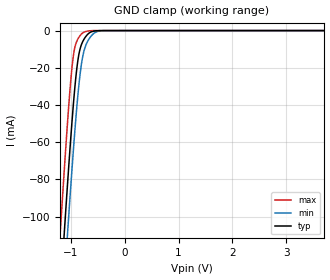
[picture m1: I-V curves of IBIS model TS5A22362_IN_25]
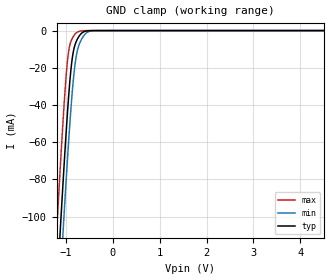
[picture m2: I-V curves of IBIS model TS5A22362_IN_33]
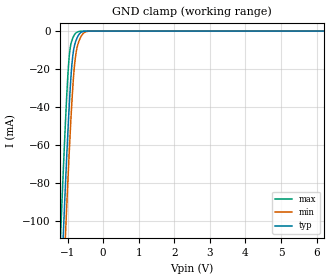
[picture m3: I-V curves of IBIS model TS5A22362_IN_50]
| TEXAS INSTRUMENTS INCORPORATED
| Standard Linear and Logic Group
| IBIS Model of TS5A22362
| 0.65-OHM DUAL SPDT ANALOG SWITCHES WITH NEGATIVE SIGNALING CAPABILITY
| This file contains package information for the following:
|  VSSOP 10-pin (DGS) package as [Component] TS5A22362_DGS
| This device can be powered at the following Vccs:
|  2.5 volt Vcc
|  3.3 volt Vcc
|  5 volt Vcc
| This file provides unique models under the [Model Selector] for each Vcc.
| For operation at a specific Vcc, select the appropriate model after each
| [Model Selector] keyword.
[IBIS Ver]   3.2
[Comment char]  |_char
[File Name]   ts5a22362.ibs
[File Rev]   1.0 | x_die
[Date]   March 22, 2009
[Source]   Data created from TI-SPICE simulations at TI-SLL.
[Notes]   The following is an IBIS list for the TS5A22362.
   Please contact sllibis@ti.com with questions and
   comments concerning SLL IBIS models.
   - FILE REV HISTORY
   - 1.0 Release IBIS file on 03/23/09.
   - Power clamp data deleted was deleted as there is no
   power-clamp diode.
   - No ground clamp current for the COM and N models
   due to negative voltages passed through the switch.
   - Non-monotonic data due to FET characteristics.
[Disclaimer] Property of Texas Instruments Incorporated.  Unauthorized
   reproduction and/or distribution is strictly prohibited.
   This product is protected under copyright law.
   Created  2009, (C) Copyright  2009, Texas Instruments
   Incorporated, All Rights Reserved
   UNLESS THERE IS A SIGNED, WRITTEN AGREEMENT TO THE
   CONTRARY, TEXAS INSTRUMENTS (TI) IS PROVIDING THE IBIS
   MODELS  AND WITHOUT ANY WARRANTY, EXPRESSED OR
   IMPLIED.  TI assumes no liability for:
   1) the accuracy of the IBIS models provided to your
   company;
   2) the proper functioning of these IBIS Models in your
   design or for any resulting applications; or
   3) infringement of patents, copyrights or intellectual
   property rights resulting from your use of these IBIS
   models.
   TI provides IBIS Models as a service to our customers.
   You and your company shall not distribute, sell or give
   these models to anyone else without prior written
   permission from TI.
   TI reserves the right to make changes to our products or
   to discontinue any semiconductor product or service
   without notice, and advises our customers to obtain the
   latest version of relevant information to verify, before
   placing orders, that the information being relied on is
   current.
   Please be aware that your receipt and use of the IBIS
   information provided shall serve as acceptance of these
   terms and conditions.  If you do not accept these terms,
   you should return or destroy the IBIS models and any
   other accompanying information immediately.
| Component TS5A22362_DGS 10-PIN VSSOP
[Component]   TS5A22362_DGS
[Manufacturer]   Texas Instruments, Inc.
[Package]
|   typ   min   max
R_pkg   4.300e-02   4.100e-02   4.700e-02
L_pkg   2.235e-09   2.157e-09   2.339e-09
C_pkg   3.350e-13   3.080e-13   3.550e-13
[Pin]   signal_name   model_name   R_pin   L_pin   C_pin
1   VP   POWER   4.700e-02   2.339e-09   3.100e-13
2   NO1   TS5A22362_N   4.300e-02   2.213e-09   3.550e-13
3   COM1   TS5A22362_COM   4.100e-02   2.157e-09   3.540e-13
4   NC1   TS5A22362_N   4.300e-02   2.213e-09   3.550e-13
5   IN1   TS5A22362_IN   4.700e-02   2.339e-09   3.100e-13
6   GND   GND   4.500e-02   2.284e-09   3.080e-13
7   IN2   TS5A22362_IN   4.100e-02   2.176e-09   3.500e-13
8   NC2   TS5A22362_N   4.100e-02   2.172e-09   3.500e-13
9   COM2   TS5A22362_COM   4.100e-02   2.176e-09   3.510e-13
10   NO2   TS5A22362_N   4.500e-02   2.284e-09   3.080e-13
[Series Switch Groups]
| Function Group States
On  1 /   | NC1-NC2->COM1-COM2 IN1-IN2, LOW
   | COM1-COM2->NC1-NC2 IN1-IN2, LOW
On  2 /   | NO1-NO2->COM1-COM2 IN1-IN2, HIGH
   | COM1-COM2->NO1-NO2 IN1-IN2, HIGH
On  1 /   | IN1-IN2, LOW
Off 2 /   | IN1-IN2, HIGH
[Series Pin Mapping]   pin_2   model_name   function_table_group
4   3   TS5A22362_N_25_S   1
| 4   3   TS5A22362_N_33_S   1
| 4   3   TS5A22362_N_50_S   1
8   9   TS5A22362_N_25_S   1
| 8   9   TS5A22362_N_33_S   1
| 8   9   TS5A22362_N_50_S   1
3   4   TS5A22362_COM_25_S   1
| 3   4   TS5A22362_COM_33_S   1
| 3   4   TS5A22362_COM_50_S   1
9   8   TS5A22362_COM_25_S   1
| 9   8   TS5A22362_COM_33_S   1
| 9   8   TS5A22362_COM_50_S   1
2   3   TS5A22362_N_25_S   2
| 2   3   TS5A22362_N_33_S   2
| 2   3   TS5A22362_N_50_S   2
10   9   TS5A22362_N_25_S   2
| 10   9   TS5A22362_N_33_S   2
| 10   9   TS5A22362_N_50_S   2
3   2   TS5A22362_COM_25_S   2
| 3   2   TS5A22362_COM_33_S   2
| 3   2   TS5A22362_COM_50_S   2
9   10   TS5A22362_COM_25_S   2
| 9   10   TS5A22362_COM_33_S   2
| 9   10   TS5A22362_COM_50_S   2
| Model TS5A22362_IN
[Model Selector]   TS5A22362_IN
TS5A22362_IN_25   2.5 volt Vcc
TS5A22362_IN_33   3.3 volt Vcc
TS5A22362_IN_50   5 volt Vcc
| Model TS5A22362_N
[Model Selector]   TS5A22362_N
TS5A22362_N_25   2.5 volt Vcc
TS5A22362_N_33   3.3 volt Vcc
TS5A22362_N_50   5 volt Vcc
| Model TS5A22362_N_S
[Model Selector]   TS5A22362_N_S
TS5A22362_N_25_S   2.5 volt Vcc
TS5A22362_N_33_S   3.3 volt Vcc
TS5A22362_N_50_S   5 volt Vcc
| Model TS5A22362_COM
[Model Selector]   TS5A22362_COM
TS5A22362_COM_25   2.5 volt Vcc
TS5A22362_COM_33   3.3 volt Vcc
TS5A22362_COM_50   5 volt Vcc
| Model TS5A22362_COM_S
[Model Selector]   TS5A22362_COM_S
TS5A22362_COM_25_S   2.5 volt Vcc
TS5A22362_COM_33_S   3.3 volt Vcc
TS5A22362_COM_50_S   5 volt Vcc
[Model]   TS5A22362_N_25_S
Model_type  Series_switch
| variable   typ   min   max
C_comp   0   0   0
[Temperature Range]   40   100   -40
| Ambient temperature   25   85   -40
[Voltage range]   2.5   2.3   2.7
[On]
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[Off]
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[Model]   TS5A22362_N_33_S
Model_type  Series_switch
| variable   typ   min   max
C_comp   0   0   0
[Temperature Range]   40   100   -40
| Ambient temperature   25   85   -40
[Voltage range]   3.3   3   3.6
[On]
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[Off]
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[Model]   TS5A22362_N_50_S
Model_type  Series_switch
| variable   typ   min   max
C_comp   0   0   0
[Temperature Range]   40   100   -40
| Ambient temperature   25   85   -40
[Voltage range]   5   4.5   5.5
[On]
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[Off]
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[Model]   TS5A22362_COM_25_S
Model_type  Series_switch
| variable   typ   min   max
C_comp   0   0   0
[Temperature Range]   40   100   -40
| Ambient temperature   25   85   -40
[Voltage range]   2.5   2.3   2.7
[On]
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[Off]
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[Model]   TS5A22362_COM_33_S
Model_type  Series_switch
| variable   typ   min   max
C_comp   0   0   0
[Temperature Range]   40   100   -40
| Ambient temperature   25   85   -40
[Voltage range]   3.3   3   3.6
[On]
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[Off]
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[Model]   TS5A22362_COM_50_S
Model_type  Series_switch
| variable   typ   min   max
C_comp   0   0   0
[Temperature Range]   40   100   -40
| Ambient temperature   25   85   -40
[Voltage range]   5   4.5   5.5
[On]
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[Off]
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| Models and submodels in the file (15): TS5A22362_IN_25 (Input), TS5A22362_IN_33 (Input), TS5A22362_IN_50 (Input), TS5A22362_N_25_S (Series_switch), TS5A22362_N_25 (Terminator), TS5A22362_N_33_S (Series_switch), TS5A22362_N_33 (Terminator), TS5A22362_N_50_S (Series_switch), TS5A22362_N_50 (Terminator), TS5A22362_COM_25_S (Series_switch), TS5A22362_COM_25 (Terminator), TS5A22362_COM_33_S (Series_switch), TS5A22362_COM_33 (Terminator), TS5A22362_COM_50_S (Series_switch), TS5A22362_COM_50 (Terminator)
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[Model]   TS5A22362_IN_25
Model_type  Input
Vinl=0.6
Vinh=1.4
| variable   typ   min   max
C_comp   2.05pF   1.68pF   2.72pF
[Temperature Range]   40   100   -40
| Ambient temperature   25   85   -40
[Voltage range]   2.5   2.3   2.7
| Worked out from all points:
|   GND clamp passes 1 mA (typ) near -0.64 V on its own axis
[GND Clamp]
| TS5A22362_IN_25
|   Voltage   I(typ)   I(min)   I(max)
-2.5V     -779mA     -802.6mA   -750.6mA
-1.21V    -147.9mA   -175mA     -114.1mA
-1.185V   -136.5mA   -163.6mA   -102.6mA
-1.125V   -109.5mA   -136.5mA   -75.72mA
-1.055V   -79.15mA   -105.8mA   -46.21mA
-1V       -56.72mA   -82.65mA   -25.99mA
-955mV    -39.95mA   -64.64mA   -13.73mA
-865mV    -15.04mA   -33.13mA   -4.26mA
-765mV    -5.08mA    -11.91mA   -969.2uA
-625mV    -721.4uA   -2.983mA   -61.83uA
-440mV    -14.26uA   -138.9uA   -114.1nA
5V        57.44pA    4.993nA    32.5pA
[Model]   TS5A22362_IN_33
Model_type  Input
Vinl=0.8
Vinh=1.4
| variable   typ   min   max
C_comp   1.98pF   1.59pF   2.73pF
[Temperature Range]   40   100   -40
| Ambient temperature   25   85   -40
[Voltage range]   3.3   3   3.6
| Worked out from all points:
|   GND clamp passes 1 mA (typ) near -0.64 V on its own axis
[GND Clamp]
| TS5A22362_IN_33
|   Voltage   I(typ)   I(min)   I(max)
-3.3V     -1.181A    -1.203A    -1.155A
-1.21V    -147.9mA   -175mA     -114.1mA
-1.19V    -138.8mA   -165.9mA   -104.9mA
-1.12V    -107.3mA   -134.3mA   -73.53mA
-1.06V    -81.26mA   -108mA     -48.21mA
-950mV    -38.21mA   -62.71mA   -12.73mA
-855mV    -13.32mA   -30.21mA   -3.774mA
-800mV    -7.229mA   -17.21mA   -1.716mA
-740mV    -3.89mA    -9.301mA   -651.4uA
-595mV    -429.2uA   -2.027mA   -26.72uA
-405mV    -5.598uA   -67.63uA   -27.26nA
6.6V      76.47pA    6.838nA    42.9pA
[Model]   TS5A22362_IN_50
Model_type  Input
Vinl=0.8
Vinh=2.4
| variable   typ   min   max
C_comp   1.88pF   1.47pF   2.81pF
[Temperature Range]   40   100   -40
| Ambient temperature   25   85   -40
[Voltage range]   5   4.5   5.5
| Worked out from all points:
|   GND clamp passes 1 mA (typ) near -0.64 V on its own axis
[GND Clamp]
| TS5A22362_IN_50
|   Voltage   I(typ)   I(min)   I(max)
-5V       -2.042A    -2.059A    -2.021A
-1.19V    -138.8mA   -165.9mA   -104.9mA
-1.11V    -102.9mA   -129.9mA   -69.18mA
-1.06V    -81.26mA   -108mA     -48.21mA
-960mV    -41.72mA   -66.59mA   -14.82mA
-895mV    -21.59mA   -42.73mA   -6.039mA
-830mV    -9.948mA   -23.61mA   -2.712mA
-780mV    -5.912mA   -13.91mA   -1.237mA
-710mV    -2.707mA   -7.034mA   -396.8uA
-560mV    -224.9uA   -1.2mA     -9.122uA
-375mV    -2.411uA   -35.36uA   -7.715nA
10V       123.7pA    12.52nA    65pA
